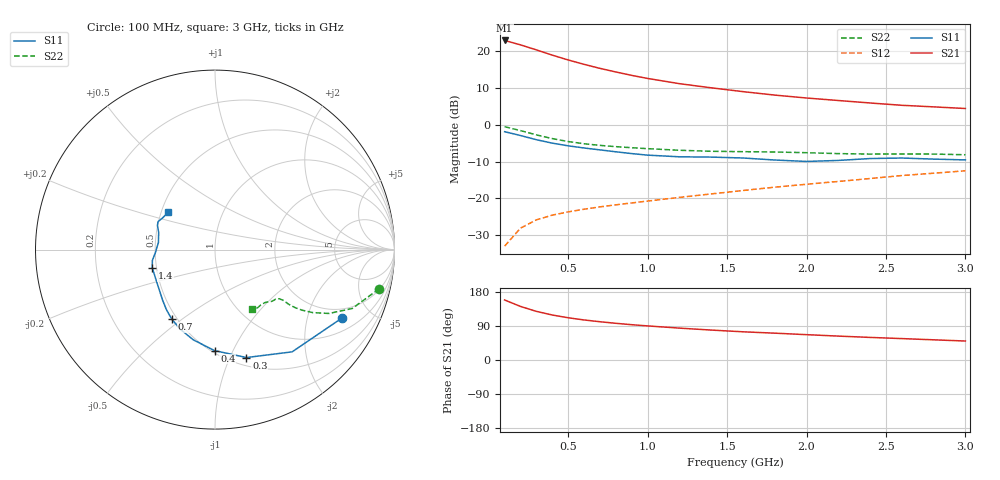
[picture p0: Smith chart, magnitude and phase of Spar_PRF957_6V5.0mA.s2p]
! Filename:  PRF957M.S2P  Version:  3.0
! NXP part #:  PRF957  Date:  Nov 1998
! Bias condition:  Vce=6V, Ic=5mA
#  MHz  S  MA  R 50
! Freq  S11  S21  S12  S22
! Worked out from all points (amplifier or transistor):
!   20 points, 100 MHz to 3 GHz, reference 50 ohm
!   highest |S21| = 22.8 dB at 100 MHz (marker M1)
!   |S21| within 3 dB of that: start of sweep to 331.1 MHz
!   unconditionally stable (mu >= 1): 1.473 GHz to end of sweep
!   at 400 MHz: K = 0.47, MSG = 21.7 dB, |S12| = -24.5 dB
!   at 1.2 GHz: K = 0.96, MSG = 15.4 dB, |S12| = -19.7 dB
!   at 3 GHz: K = 1.05, MAG = 7.1 dB, |S12| = -12.5 dB
!   lowest NFmin = 0.97 dB at 500 MHz
!   S11 on the Smith chart (normalised r, x): 100 MHz: 1.54, -3.31; 300 MHz: 0.58, -1.15; 400 MHz: 0.52, -0.85; 700 MHz: 0.47, -0.46; 1.4 GHz: 0.47, -0.11; 3 GHz: 0.54, +0.25
100  0.8043 -28.2  13.87 158.4  0.02259 75.4  0.9401 -13.4
200  0.7136 -53.0  12.08 141.3  0.03964 65.2  0.8319 -23.2
300  0.6263 -73.8  10.33 128.3  0.0513 59.1  0.728 -29.3
400  0.5626 -90.3  8.769 118.7  0.05945 56.1  0.6483 -32.8
500  0.5175 -103.4  7.542 111.5  0.06591 55.2  0.5915 -34.8
600  0.4839 -113.7  6.58 105.7  0.07157 55.3  0.552 -35.9
700  0.4558 -122.0  5.802 100.9  0.07697 56.0  0.5246 -36.4
800  0.4295 -129.2  5.185 96.8  0.08202 57.1  0.5043 -36.6
900  0.4061 -135.9  4.662 93.2  0.08703 58.4  0.4877 -36.6
1000  0.3871 -142.4  4.239 89.9  0.09233 59.8  0.4737 -36.7
1200  0.3674 -154.7  3.6 84.1  0.1035 62.1  0.4505 -37.4
1400  0.364 -163.9  3.164 79.0  0.1154 64.2  0.4364 -39.2
1600  0.354 -170.3  2.807 74.4  0.1283 66.2  0.4312 -41.2
1800  0.3323 -177.2  2.521 70.8  0.1423 67.9  0.4268 -42.6
2000  0.3178 172.8  2.301 66.9  0.156 69.2  0.4175 -44.0
2200  0.328 163.0  2.128 63.1  0.1702 70.2  0.4058 -46.6
2400  0.3479 157.2  1.971 59.6  0.1864 70.8  0.4 -50.2
2600  0.3537 153.8  1.833 56.5  0.2048 71.2  0.4015 -53.4
2800  0.3419 149.3  1.745 53.3  0.2201 71.7  0.4 -55.7
3000  0.3335 141.6  1.659 50.1  0.2374 72.2  0.3916 -58.2
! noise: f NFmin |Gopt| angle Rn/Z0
500  0.97  0.33  28  0.19
800  1.17  0.28  64  0.21
900  1.2  0.34  52  0.22
1000  1.26  0.24  74  0.26
1500  1.31  0.32  113  0.18
2000  1.71  0.29  178  0.14
